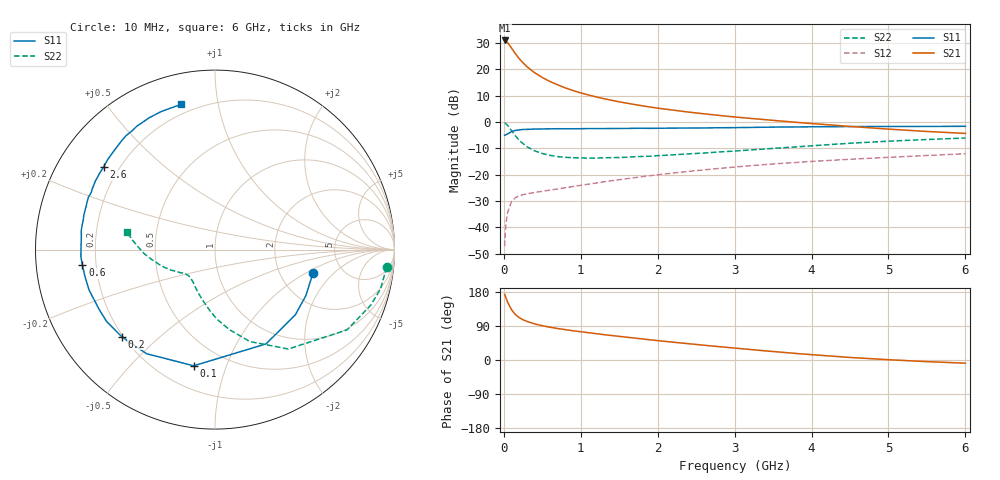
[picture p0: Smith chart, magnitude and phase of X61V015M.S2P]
! SIEMENS Small Signal Semiconductors
! BFP193W
! Si NPN RF Bipolar Junction Transistor in SOT343
! VCE = 1 V  IC = 15 mA
! Common Emitter S-Parameters:  April 1994
# GHz  S  MA  R  50
!  f  S11  S21  S12  S22
! GHz  MAG  ANG  MAG  ANG  MAG  ANG  MAG  ANG
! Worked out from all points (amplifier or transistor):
!   40 points, 10 MHz to 6 GHz, reference 50 ohm
!   highest |S21| = 31.0 dB at 10 MHz (marker M1)
!   |S21| within 3 dB of that: start of sweep to 102.4 MHz
!   unconditionally stable (mu >= 1): 980.5 MHz to 5.5 GHz
!   at 200 MHz: K = 0.31, MSG = 26.0 dB, |S12| = -28.0 dB
!   at 1.5 GHz: K = 1.14, MAG = 12.5 dB, |S12| = -21.9 dB
!   at 6 GHz: K = 0.98, MSG = 3.9 dB, |S12| = -12.0 dB
!   S11 on the Smith chart (normalised r, x): 10 MHz: 3.08, -1.16; 100 MHz: 0.34, -0.77; 200 MHz: 0.19, -0.38; 600 MHz: 0.15, -0.06; 2.6 GHz: 0.14, +0.32; 6 GHz: 0.15, +0.78
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0.01  0.5615 -13.3  35.46 173.3  0.0044 86.5  0.9616 -5.8
0.02  0.5675 -26.8  35.19 168.2  0.0088 79.4  0.948 -13.3
0.03  0.5766 -39.1  34.44 162.7  0.0128 75.5  0.9216 -19.6
0.05  0.5974 -61.6  32.1 152.1  0.0195 65.9  0.8611 -31.3
0.1  0.6582 -100.4  25.4 132.7  0.031 49.5  0.6881 -53.6
0.15  0.694 -123.3  19.91 119.9  0.0366 41.1  0.5482 -69.2
0.2  0.7111 -137.0  15.98 111.9  0.0398 37.0  0.4522 -79.9
0.25  0.7246 -146.3  13.32 106.1  0.0419 34.1  0.3891 -88.2
0.3  0.7265 -152.8  11.26 101.9  0.0434 33.2  0.3408 -94.9
0.4  0.737 -162.3  8.663 95.3  0.046 32.8  0.2845 -105.0
0.5  0.7397 -168.4  7.02 90.4  0.0485 34.6  0.2531 -112.6
0.6  0.7441 -173.3  5.882 86.5  0.0511 36.0  0.2333 -118.6
0.8  0.7466 179.6  4.455 80.1  0.0567 39.5  0.214 -126.6
1.1  0.7528 171.8  3.275 72.0  0.0663 43.7  0.2069 -134.4
1.3  0.7526 167.1  2.78 66.9  0.0732 45.8  0.2092 -137.6
1.6  0.758 160.9  2.283 60.0  0.0841 47.9  0.215 -141.2
2.2  0.7678 150.4  1.687 47.0  0.1075 48.9  0.2387 -148.3
2.6  0.7727 143.5  1.436 39.0  0.1237 48.1  0.2582 -152.9
3.2  0.7906 133.9  1.177 27.8  0.148 45.8  0.2956 -160.0
4.5  0.8211 116.4  0.827 6.7  0.1967 38.3  0.3963 -176.9
5.5  0.8262 107.6  0.663 -4.3  0.232 32.4  0.4665 173.0
6  0.8304 103.2  0.609 -8.4  0.2503 29.7  0.4976 168.9
